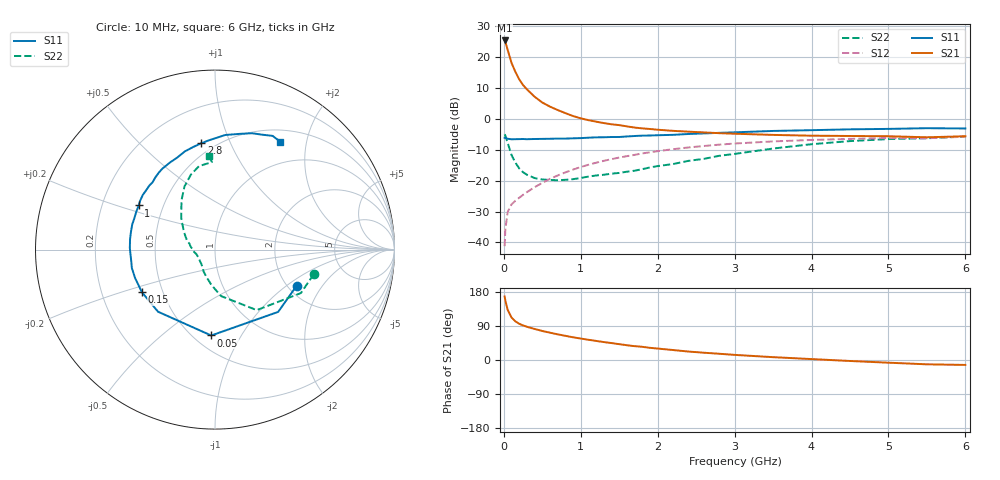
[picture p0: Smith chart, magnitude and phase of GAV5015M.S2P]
! Infineon Technologies  Discrete & RF Semiconductors
! BF775
! Si NPN RF Bipolar Junction Transistor in SOT23
! VCE = 0.5 V  IC = 15 mA
! Common Emitter S-Parameters:  May  1996
# GHz  S  MA  R  50
!  f  S11  S21  S12  S22
! GHz  MAG  ANG  MAG  ANG  MAG  ANG  MAG  ANG
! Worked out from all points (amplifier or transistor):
!   36 points, 10 MHz to 6 GHz, reference 50 ohm
!   highest |S21| = 25.5 dB at 10 MHz (marker M1)
!   |S21| within 3 dB of that: start of sweep to 49.27 MHz
!   unconditionally stable (mu >= 1): start of sweep to 18.96 MHz; 77.9 MHz to end of sweep
!   at 250 MHz: K = 1.89, MAG = 12.3 dB, |S12| = -24.6 dB
!   at 1.4 GHz: K = 2.12, MAG = -0.4 dB, |S12| = -13.0 dB
!   at 6 GHz: K = 1.18, MAG = -2.5 dB, |S12| = -5.7 dB
!   S11 on the Smith chart (normalised r, x): 10 MHz: 2.23, -1.19; 50 MHz: 0.61, -0.75; 150 MHz: 0.38, -0.23; 1 GHz: 0.36, +0.24; 2.8 GHz: 0.43, +0.78; 6 GHz: 0.66, +1.56
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0.01  0.4975 -23.9  18.77 167.7  0.0087 75.8  0.5668 -14.0
0.02  0.4943 -44.6  17.79 156.6  0.0163 68.2  0.5367 -26.8
0.05  0.479 -92.5  13.19 132.3  0.0312 52.9  0.4097 -55.4
0.1  0.4696 -132.5  8.121 112.0  0.0413 44.2  0.2611 -82.6
0.15  0.4715 -149.8  5.812 102.0  0.0475 44.5  0.1963 -96.2
0.2  0.4726 -160.6  4.394 95.6  0.0529 47.3  0.1586 -107.7
0.25  0.4745 -167.5  3.547 91.1  0.0591 49.6  0.1374 -117.7
0.3  0.4711 -172.3  3.031 87.7  0.0654 52.1  0.1251 -122.6
0.4  0.4746 178.9  2.296 81.9  0.0786 55.4  0.1105 -133.4
0.5  0.4768 173.0  1.851 76.6  0.0923 57.5  0.1047 -144.1
0.6  0.4787 167.8  1.588 72.1  0.1073 58.4  0.1031 -150.6
0.8  0.482 158.8  1.246 63.8  0.1366 58.5  0.1035 -159.6
1  0.4907 149.9  1.026 56.6  0.1666 57.4  0.111 -169.7
1.1  0.4983 146.8  0.959 53.4  0.1815 56.3  0.1168 -173.4
1.3  0.5065 139.1  0.86 47.3  0.2103 54.0  0.125 179.2
1.7  0.5308 126.2  0.727 36.5  0.2626 48.4  0.1454 167.2
2.2  0.5543 112.3  0.643 26.3  0.3244 40.5  0.1865 153.9
2.8  0.5971 97.4  0.59 16.5  0.3846 30.7  0.2536 137.7
3.5  0.6411 84.9  0.553 7.5  0.4337 19.8  0.3326 124.1
4.5  0.6805 72.3  0.531 -2.6  0.4767 6.4  0.4389 107.8
5.5  0.7103 63.1  0.506 -11.4  0.4882 -5.4  0.4881 92.0
6  0.7025 59.0  0.526 -13.0  0.5166 -8.8  0.5219 93.6
